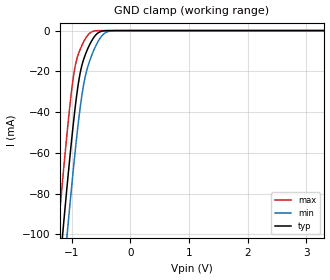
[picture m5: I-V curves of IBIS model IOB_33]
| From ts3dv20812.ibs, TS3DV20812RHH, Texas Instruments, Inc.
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[Model]   IOB_33
Model_type  Terminator
| variable   typ   min   max
C_comp   2.33pF   2.05pF   2.59pF
| C_tri-state   2.33pF   2.05pF   2.59pF
[Temperature Range]   40   100   -40
| Ambient temperature   25   85   -40
[Voltage range]   3.3   3   3.6
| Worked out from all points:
|   GND clamp passes 1 mA (typ) near -0.54 V on its own axis
[GND Clamp]
| TS3DV20812_IOB_33
|   Voltage   I(typ)   I(min)   I(max)
-3.3V     -888.4mA   -907.4mA   -874.2mA
-1.24V    -126.8mA   -151.7mA   -99.9mA
-1.145V   -96.02mA   -120.5mA   -69.36mA
-1.07V    -72.79mA   -96.66mA   -46.83mA
-955mV    -40.56mA   -62.46mA   -19.2mA
-880mV    -24.29mA   -42.86mA   -10.81mA
-810mV    -15.16mA   -28.36mA   -6.138mA
-745mV    -9.978mA   -19.47mA   -2.885mA
-665mV    -5.178mA   -12.42mA   -679.8uA
-490mV    -327.2uA   -2.684mA   -3.494uA
-330mV    -5.418uA   -173uA     -5.364nA
3.3V      852.5pA    392.1nA    32.38pA
